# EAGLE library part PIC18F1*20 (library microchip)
18/20/28-Pin High-Performance, Enhanced Flash Microcontrollers with 10-bit A/D and nanoWatt Technology Source: ww1.microchip.com/downloads/en/DeviceDoc/39605c.pdf
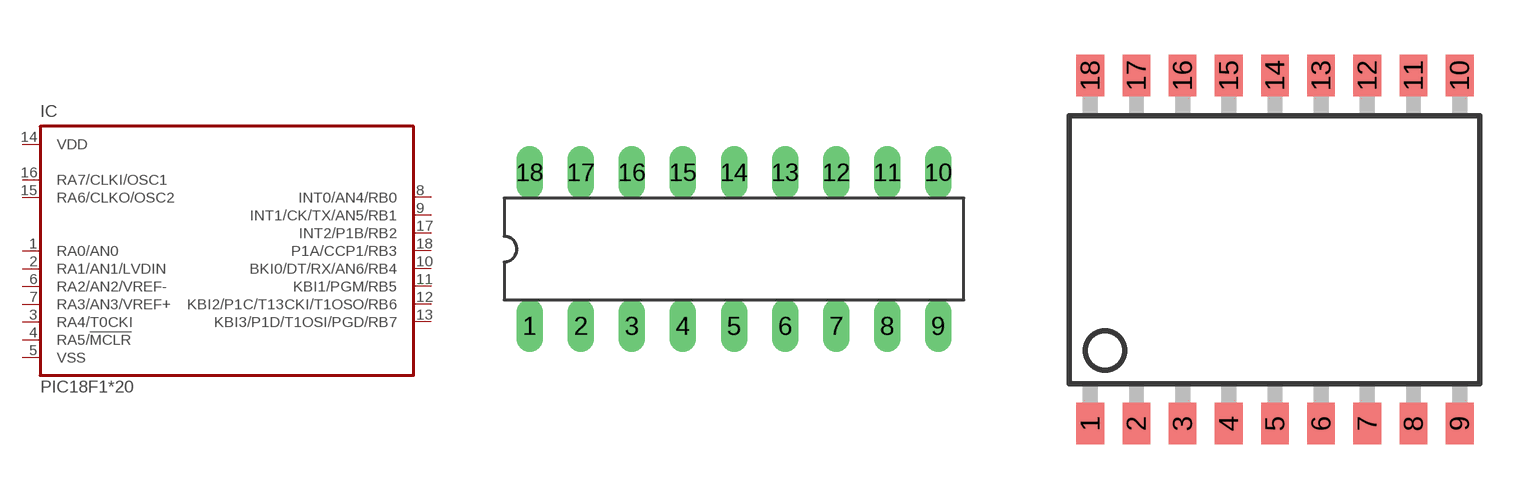
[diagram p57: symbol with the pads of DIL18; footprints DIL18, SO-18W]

Designator prefix IC

## PIC18F1220P (MF: MICROCHIP; MPN: PIC18F1220-I/P; OC_FARNELL: 9761977; OC_NEWARK: 92C2429)  [DIL18]
1  RA0/AN0
2  RA1/AN1/LVDIN
3  RA4/T0CKI
4  RA5/!MCLR  in
5  VSS  pwr
6  RA2/AN2/VREF-
7  RA3/AN3/VREF+
8  INT0/AN4/RB0
9  INT1/CK/TX/AN5/RB1
10  BKI0/DT/RX/AN6/RB4
11  KBI1/PGM/RB5
12  KBI2/P1C/T13CKI/T1OSO/RB6
13  KBI3/P1D/T1OSI/PGD/RB7
14  VDD  pwr
15  RA6/CLKO/OSC2
16  RA7/CLKI/OSC1
17  INT2/P1B/RB2
18  P1A/CCP1/RB3

## PIC18F1220SO (MF: MICROCHIP; MPN: PIC18F1220-I/SO; OC_FARNELL: 9761985; OC_NEWARK: 92C2430)  [SO-18W]
Pads as for DIL18

## Footprint DIL18 (pad centres in mm)
Dual In Line package type P
drill 0.813 long: 1 -10.16,-3.81; 2 -7.62,-3.81; 3 -5.08,-3.81; 4 -2.54,-3.81; 5 0,-3.81; 6 2.54,-3.81; 7 5.08,-3.81; 8 7.62,-3.81; 9 10.16,-3.81; 10 10.16,3.81; 11 7.62,3.81; 12 5.08,3.81; 13 2.54,3.81; 14 0,3.81; 15 -2.54,3.81; 16 -5.08,3.81; 17 -7.62,3.81; 18 -10.16,3.81

## Footprint SO-18W (pad centres in mm)
Small Outline Wide Plastic Gull Wing 300-mil body, package type SO
smd 0.762 x 1.143: 1 -5.08,-4.788; 2 -3.81,-4.788; 3 -2.54,-4.788; 4 -1.27,-4.788; 5 0,-4.788; 6 1.27,-4.788; 7 2.54,-4.788; 8 3.81,-4.788; 9 5.08,-4.788; 10 5.08,4.788; 11 3.81,4.788; 12 2.54,4.788; 13 1.27,4.788; 14 0,4.788; 15 -1.27,4.788; 16 -2.54,4.788; 17 -3.81,4.788; 18 -5.08,4.788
